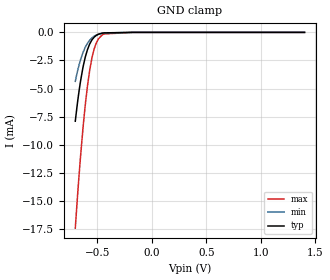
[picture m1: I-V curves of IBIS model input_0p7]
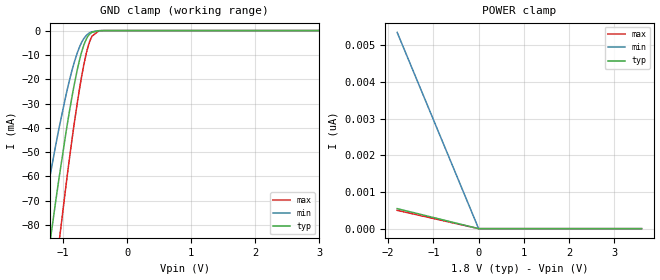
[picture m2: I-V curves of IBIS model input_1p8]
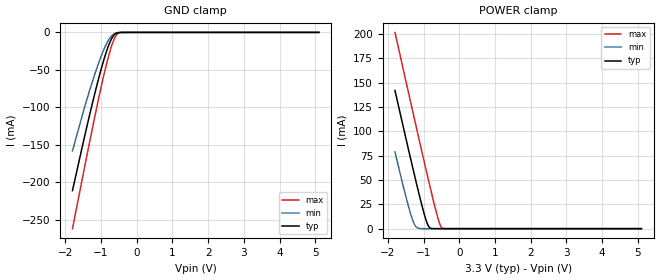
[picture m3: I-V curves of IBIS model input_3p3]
|Texas Instruments Incorporated
| 8-Bit Dual-Supply Bus Transceiver With Configurable Voltage Translation and
| 3-State Outputs
[IBIS Ver]   4.2
[File name]   sn74axc8t245.ibs
[Date]   03/06/2020
[File Rev]   1.1
[Source]
| Texas Instruments Incorporated.
| Analog-eLab Design Center, HPA
| 12500 TI Blvd
| Dallas, TX -75243
[Notes]
| Rev 1.1: 03/06/2020
| - Added input_1p8 and io_1p8 model.
| Rev 1.0: 06/08/2017
| - Initial version of the model
| - Model generated from simulations in SPECTRE
| - Model matched to SPICE simulation
| - C_comp although listed in numerical order of value are
|   obtained from varying PVT conditions. For PVT conditions for
|   each specific value refer the buffer description under
|   respective [Model]. IBIS model user is responsible for using
|   appropriate C_comp to simulate for Signal Integrity.
[Disclaimer]
| This model is designed as an aid for customers of Texas Instruments.
| TI and its licensors and suppliers make no warranties, either expressed
| or implied, with respect to this  model, including the warranties of
| merchantability or fitness for a particular purpose. The model is
| provided solely on an "as is" basis. The entire risk as to its quality
| and performance is with the customer.
[Copyright]
(C) Copyright 2017 Texas Instruments Incorporated.All rights reserved.
|   SN74AXC8T245PW
| Marketing part#   Digital Voltage Range   Package-type   #pins
| SN74AXC8T245PW   0.65V-3.6V   TSSOP   24
[Component]   SN74AXC8T245PW
[Manufacturer]  TI
[Package]   |24 TSSOP - PW package
|   typ   min   max
R_pkg   0.1143375   0.06811   0.12769
L_pkg   3.405334167nH   2.85598nH   4.17092nH
C_pkg   0.565412083pF   0.46044pF   0.71557pF
[Pin]  signal_name model_name   R_pin   L_pin   C_pin
1   VCCA   power   0.06958   3.86966nH   0.71557pF
2   DIR1   input   0.12094   3.80225nH   0.66679pF
3   A1   io   0.12769   3.54754nH   0.57242pF
4   A2   io   0.12362   3.25170nH   0.50771pF
5   A3   io   0.11601   3.02250nH   0.49462pF
6   A4   io   0.10931   2.86990nH   0.46105pF
7   A5   io   0.10845   2.85719nH   0.46044pF
8   A6   io   0.11376   2.99109nH   0.49241pF
9   A7   io   0.11998   3.20023nH   0.50408pF
10   A8   io   0.12312   3.48368nH   0.56447pF
11   DIR2   input   0.12091   3.81199nH   0.66374pF
12   GND   gnd   0.11675   4.13953nH   0.67876pF
13   GND   gnd   0.06811   3.82650nH   0.71298pF
14   B8   io   0.12091   3.81016nH   0.66711pF
15   B7   io   0.12766   3.55445nH   0.57259pF
16   B6   io   0.12359   3.25719nH   0.50787pF
17   B5   io   0.11599   3.02618nH   0.49474pF
18   B4   io   0.10929   2.87119nH   0.46118pF
19   B3   io   0.10845   2.85598nH   0.46051pF
20   B2   io   0.11377   2.98788nH   0.49236pF
21   B1   io   0.12   3.19513nH   0.50408pF
22   nOE   input   0.12314   3.47698nH   0.56494pF
23   VCCB   power   0.12375   3.84820nH   0.66804pF
24   VCCB   power   0.11932   4.17092nH   0.68143pF
|   SN74AXC8T245RHL
| Marketing part#   Digital Voltage Range   Package-type   #pins
| SN74AXC8T245RHL   0.65V-3.6V   YQFN   24
[Component]   SN74AXC8T245RHL
[Manufacturer]  TI
[Package]   |24 YQFN - RHL package
|   typ   min   max
R_pkg   0.085   0.058   0.116
L_pkg   1.593n   1.101n   2.229n
C_pkg   0.258p   0.219p   0.337p
[Pin]  signal_name model_name   R_pin   L_pin   C_pin
1   VCCA   power   0.0589   1.5334n   0.3373p
2   DIR1   input   0.1148   2.1925n   0.2676p
3   A1   io   0.0984   1.7889n   0.2917p
4   A2   io   0.0841   1.4994n   0.2570p
5   A3   io   0.0723   1.2607n   0.2333p
6   A4   io   0.0655   1.1245n   0.2200p
7   A5   io   0.0637   1.1101n   0.2185p
8   A6   io   0.0688   1.2432n   0.2289p
9   A7   io   0.0788   1.4543n   0.2506p
10   A8   io   0.0925   1.7374n   0.2753p
11   DIR2   input   0.1138   2.1938n   0.2623p
12   GND   gnd   0.1074   2.0415n   0.2530p
13   GND   gnd   0.0585   1.5096n   0.3326p
14   B8   io   0.1153   2.1253n   0.2676p
15   B7   io   0.0992   1.7605n   0.2916p
16   B6   io   0.0837   1.4781n   0.2571p
17   B5   io   0.0716   1.2733n   0.2332p
18   B4   io   0.0645   1.1262n   0.2200p
19   B3   io   0.0636   1.1010n   0.2188p
20   B2   io   0.0699   1.2254n   0.2290p
21   B1   io   0.0807   1.4310n   0.2511p
22   nOE   input   0.0943   1.7202n   0.2780p
23   VCCB   power   0.1164   2.2294n   0.2692p
24   VCCB   power   0.1093   2.0732n   0.2573p
|   SN74AXC8T245RJW
| Marketing part#   Digital Voltage Range   Package-type   #pins
| SN74AXC8T245RJW   0.65V-3.6V   uQFN   24
[Component]   SN74AXC8T245RJW
[Manufacturer]  TI
[Package]   |24 uQFN - RKT package
|   typ   min   max
R_pkg   0.078075   0.04588   0.12141
L_pkg   0.978537917nH   0.60336nH   1.54474nH
C_pkg   0.304233333pF   0.23351pF   0.36249pF
[Pin]  signal_name model_name   R_pin   L_pin   C_pin
1   DIR1   input   0.11918   1.51673nH   0.27692pF
2   A1   io   0.10353   1.29938nH   0.30726pF
3   A2   io   0.08751   1.07368nH   0.36249pF
4   A3   io   0.07203   0.86586nH   0.33880pF
5   A4   io   0.05935   0.69679nH   0.32139pF
6   A5   io   0.0523   0.60336nH   0.31235pF
7   A6   io   0.05388   0.62418nH   0.31443pF
8   A7   io   0.06332   0.74959nH   0.32669pF
9   A8   io   0.07633   0.93332nH   0.25699pF
10   DIR2   input   0.09587   1.19534nH   0.23351pF
11   GND   gnd   0.08919   1.06264nH   0.27090pF
12   GND   gnd   0.04588   0.78601nH   0.30916pF
13   B8   io   0.0958   1.19956nH   0.23938pF
14   B7   io   0.08139   1.00661nH   0.26883pF
15   B6   io   0.06751   0.81220nH   0.33269pF
16   B5   io   0.05632   0.66473nH   0.31784pF
17   B4   io   0.05189   0.60699nH   0.31231pF
18   B3   io   0.05639   0.66565nH   0.31794pF
19   B2   io   0.06763   0.81366nH   0.33284pF
20   B1   io   0.0824   1.01033nH   0.35462pF
21   nOE   input   0.09804   1.22986nH   0.28985pF
22   VCCB   power   0.12141   1.54474nH   0.26570pF
23   VCCB   power   0.1169   1.43698nH   0.29681pF
24   VCCA   power   0.05975   1.08672nH   0.34190pF
|   Model Selectors
[Model Selector] input
input_0p7   0.7V   digital Input
input_1p8   1.8V   digital Input
input_3p3   3.3V   digital Input
[Model Selector] io
io_0p7   0.7V   digital I/O
io_1p8   1.8V   digital I/O
io_3p3   3.3V   digital I/O
| Models and submodels in the file (6): input_0p7 (Input), input_1p8 (Input), input_3p3 (Input), io_0p7 (I/O), io_1p8 (I/O), io_3p3 (I/O)
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|   input_0p7 Model
[Model]   input_0p7
Model_type   Input
Vinl = 0.21
Vinh = 0.49
|   typ   min   max
C_comp   7.40696E-13   6.45127E-13   8.98734E-13
[Model spec]
|subparameter
Vinl   0.21   0.195   0.225
Vinh   0.49   0.455   0.525
| Where Nom  PVT is Nominal Process, 0.7V, 27C
|   Fast PVT is Strong Process,  0.75V, -40C
|   Slow PVT is Weak Process,   0.65, 130C
[Voltage Range]   0.7   0.65   0.75
|Junction Temperature
[Temperature Range]   27   130   -40
[Power Clamp Reference]   0.7   0.65   0.75
[GND Clamp Reference]   0   0   0
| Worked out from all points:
|   GND clamp passes 1 mA (typ) near -0.57 V on its own axis
[GND Clamp]
|   Voltage   I(typ)   I(min)   I(max)
-700mV    -7.896mA   -4.354mA   -17.4mA
-676.9mV  -6.033mA   -3.335mA   -14.2mA
-651.7mV  -4.329mA   -2.43mA    -11.02mA
-624.4mV  -2.873mA   -1.673mA   -7.992mA
-588.7mV  -1.545mA   -978.4uA   -4.797mA
-567.7mV  -1.026mA   -696.2uA   -3.358mA
-548.8mV  -691.6uA   -504.6uA   -2.342mA
-527.8mV  -434.7uA   -346.8uA   -1.503mA
-487.9mV  -168.3uA   -161.7uA   -574.9uA
-454.3mV  -71.1uA    -80.61uA   -230.7uA
-175mV    -4.456nA   -77.57nA   0A
1.4V      0A         0A         0A
[POWER Clamp]
|   Voltage   I(typ)   I(min)   I(max)
-700mV    0A         0A         0A
0V        0A         0A         0A
1.4V      0A         0A         0A
|   input_1p8 Model
[Model]   input_1p8
Model_type   Input
Vinl = 0.7
Vinh = 1.6
|   typ   min   max
C_comp   1.392pf   0.843pf   1.994pF
| Where Nom  PVT is Nominal Process, 1.8V,  27C
|   Fast PVT is Strong Process,  1.98V, -40C
|   Slow PVT is Weak Process,   1.62V, 130C
[Voltage Range]   1.8   1.62   1.98
|Junction Temperature
[Temperature Range]   27   130   -40
[Power Clamp Reference]   1.8   1.62   1.98
[GND Clamp Reference]   0   0   0
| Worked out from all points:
|   GND clamp passes 1 mA (typ) near -0.56 V on its own axis
[GND Clamp]
|   Voltage   I(typ)   I(min)   I(max)
-1.8V     -210.9mA   -157.9mA   -261.6mA
-1.319V   -109.8mA   -77.26mA   -146mA
-1.206V   -87.46mA   -60.12mA   -119.6mA
-1.12V    -71.04mA   -47.78mA   -99.81mA
-1.066V   -61.14mA   -40.45mA   -87.72mA
-952.2mV  -41.52mA   -26.26mA   -63.25mA
-903.6mV  -33.72mA   -20.8mA    -53.27mA
-779.4mV  -16.26mA   -9.28mA    -30.01mA
-676.8mV  -6.025mA   -3.331mA   -14.19mA
-579.6mV  -1.299mA   -846.1uA   -4.132mA
-385.2mV  -10.15uA   -16.94uA   -26.09uA
3.6V      0A         0A         0A
[POWER Clamp]
|   Voltage   I(typ)   I(min)   I(max)
-1.8V     546.7pA    5.348nA    499.5pA
0V        0A         0A         0A
3.6V      0A         0A         0A
|   input_3p3 Model
[Model]   input_3p3
Model_type   Input
Vinl = 0.8
Vinh = 2.3
|   typ   min   max
C_comp   1.86062E-12   1.26954E-12   2.13619E-12
| Where Nom  PVT is Nominal Process, 3.3V, 27C
|   Fast PVT is Strong Process,  3.6V, -40C
|   Slow PVT is Weak Process,   3.0V, 130C
[Voltage Range]   3.3   3   3.6
|Junction Temperature
[Temperature Range]   27   130   -40
[Power Clamp Reference]   3.3   3   3.6
[GND Clamp Reference]   0   0   0
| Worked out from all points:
|   GND clamp passes 1 mA (typ) near -0.57 V on its own axis
|   POWER clamp passes 1 mA (typ) near -0.83 V on its own axis
[GND Clamp]
|   Voltage   I(typ)   I(min)   I(max)
-1.8V     -210.9mA   -157.9mA   -261.6mA
-1.49V    -144.7mA   -104.6mA   -186.5mA
-1.296V   -105.2mA   -73.69mA   -140.6mA
-1.117V   -70.54mA   -47.4mA    -99.2mA
-951.3mV  -41.37mA   -26.15mA   -63.06mA
-820.2mV  -21.52mA   -12.61mA   -37.23mA
-716.7mV  -9.415mA   -5.207mA   -19.86mA
-613.2mV  -2.39mA    -1.422mA   -6.892mA
-523.5mV  -394uA     -320.5uA   -1.365mA
-426.9mV  -33.77uA   -44.18uA   -102.3uA
-68.1mV   0A         0A         0A
5.1V      0A         0A         0A
[POWER Clamp]
|   Voltage   I(typ)   I(min)   I(max)
-1.8V     141.9mA    78.74mA    201.4mA
-1.414V   79.93mA    21.78mA    138.3mA
-1.296V   61.5mA     8.016mA    119.2mA
-1.234V   51.89mA    3.123mA    109.2mA
-1.151V   39.29mA    456.6uA    95.81mA
-985.8mV  15.65mA    4.189uA    69.3mA
-868.5mV  3.093mA    131.9nA    50.79mA
-799.5mV  400.9uA    7.757nA    40.08mA
-571.8mV  47.54nA    0A         7.669mA
-516.6mV  0A         0A         2.383mA
-468.3mV  0A         0A         390.4uA
5.1V      0A         0A         0A
